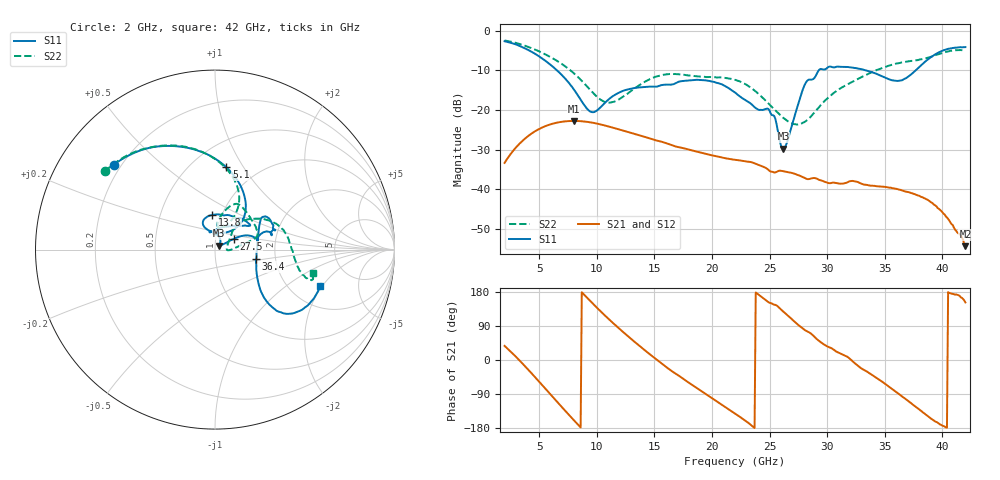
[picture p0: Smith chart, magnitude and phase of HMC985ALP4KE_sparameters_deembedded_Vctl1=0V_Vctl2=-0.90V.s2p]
!s2p File: Measurements: S11, S21, S12, S22
# GHz S dB R 50.0
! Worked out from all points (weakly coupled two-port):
!   401 points, 2 GHz to 42 GHz, reference 50 ohm
!   highest |S21| = -22.77 dB at 8 GHz (marker M1); lowest = -54.4 dB at 42 GHz (marker M2)
!   lowest |S11| = -29.8 dB at 26.2 GHz (marker M3), VSWR 1.07, Z = 52.4 + j2.26 ohm
!   |S11| at or under -10 dB: 6.546 GHz to 29.27 GHz (22.73 GHz wide, 127 % of centre); 33.35 GHz to 37.69 GHz (4.345 GHz wide, 12.2 % of centre)
!   |S22| runs from -23.7 to -2.5 dB; largest |S21 - S12| = 0.00012
!   S11 on the Smith chart (normalised r, x): 2 GHz: 0.17, +0.35; 5.1 GHz: 0.72, +0.84; 13.8 GHz: 0.90, +0.36; 27.5 GHz: 1.22, +0.15; 36.4 GHz: 1.58, -0.17; 42 GHz: 2.90, -1.91
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2  -2.66 140.1  -33.36 37.2  -33.36 37.2  -2.46 144.7
3.5  -4.10 112.3  -27.94 -7.7  -27.94 -7.7  -3.54 120.4
5.1  -6.69 82.2  -24.65 -60.7  -24.66 -60.7  -5.36 95.9
8  -14.77 45.5  -22.77 -158.5  -22.77 -158.5  -10.71 62.8
8.7  -17.86 51.8  -22.85 178.8  -22.86 178.8  -12.66 60.2
9.7  -20.56 86.0  -23.25 147.5  -23.25 147.5  -15.77 63.1
11  -17.40 114.5  -24.14 109.1  -24.15 109.0  -18.15 78.1
13.8  -14.27 95.3  -26.49 35.0  -26.49 35.0  -13.54 77.6
15.4  -13.94 73.0  -27.85 -3.4  -27.84 -3.4  -11.37 68.3
19.4  -12.52 34.6  -31.03 -88.7  -31.04 -88.7  -11.66 35.8
22  -15.60 52.2  -32.57 -141.0  -32.59 -141.0  -12.39 16.8
25  -20.20 97.8  -35.37 150.9  -35.38 151.0  -18.68 5.6
26.2  -29.80 41.7  -35.46 127.4  -35.47 127.4  -22.00 -2.4
27.5  -18.41 29.7  -36.45 92.3  -36.48 92.4  -23.60 4.7
28.1  -13.36 20.7  -37.22 78.2  -37.22 78.2  -22.92 16.9
28.7  -12.31 12.9  -37.22 66.9  -37.22 67.1  -21.29 28.8
31  -9.08 23.4  -38.56 19.3  -38.55 19.1  -14.81 49.2
33.3  -9.96 34.4  -38.87 -28.0  -38.85 -28.0  -11.29 38.9
35.4  -12.27 12.3  -39.62 -71.1  -39.60 -71.1  -8.82 24.2
36.4  -12.57 -12.8  -40.19 -93.6  -40.21 -93.9  -8.04 16.2
39.5  -5.80 -43.3  -44.35 -163.8  -44.39 -163.3  -6.07 -14.6
42  -4.14 -19.0  -54.37 151.8  -54.48 151.1  -4.98 -13.6
